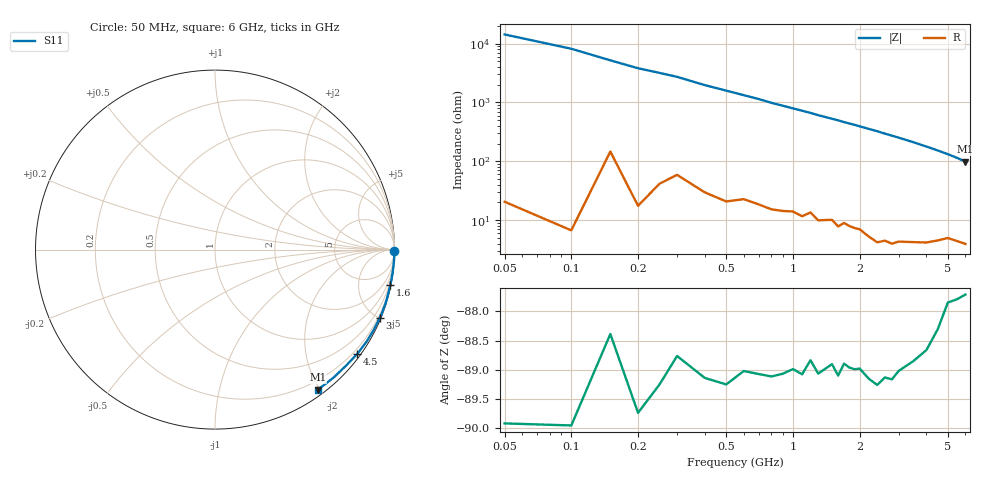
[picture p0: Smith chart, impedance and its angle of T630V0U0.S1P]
! SIEMENS Discrete & RF Semiconductors
! BAT62
! Si Schottky Diode in SOT143
! VR = 30 V
! S-Parameters:  February  1997
# GHz  S  MA  R  50
!  f  S11
! GHz  MAG  ANG
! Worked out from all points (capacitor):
!   34 points, 50 MHz to 6 GHz, reference 50 ohm
!   read as one part to ground: C = 204 fF near 50 MHz
!   lowest |Z| = 98.7 ohm at 6 GHz (marker M1)
!   S11 on the Smith chart (normalised r, x): 50 MHz: open; 1.6 GHz: 0.16, -9.93; 3 GHz: 0.09, -5.05; 4.5 GHz: 0.09, -3.06; 6 GHz: 0.08, -1.97
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0.05  1 -0.4
0.1  1 -0.7
0.15  0.9995 -1.1
0.2  0.9999 -1.5
0.3  0.9992 -2.1
0.4  0.9992 -2.9
0.5  0.9992 -3.6
0.7  0.9986 -5.0
0.8  0.9984 -5.8
1.1  0.9978 -7.9
1.2  0.997 -8.6
1.3  0.9973 -9.4
1.5  0.9964 -10.8
1.6  0.9969 -11.5
1.7  0.9959 -12.3
1.9  0.9958 -13.7
2  0.9956 -14.5
2.2  0.9959 -16.0
2.4  0.9961 -17.5
2.6  0.995 -19.2
2.8  0.9948 -20.8
3  0.9935 -22.4
3.5  0.991 -26.7
4  0.9879 -31.3
4.5  0.9827 -36.2
5  0.9755 -41.4
5.5  0.9721 -47.2
6  0.9683 -53.7
